(* Logix 5000 AddOnInstructionDefinition export MSQR_Yaskawa; software revision 17.00 *)

TYPE Yaskawa_EIP_Servo :   // Yaskawa SigmaLogic Axis Structure v2.4.0
STRUCT
   O : Yaskawa_OUT_to_Servo;
   I : Yaskawa_IN_from_Servo;
   AOI_SB : Yaskawa_AOI_Status_Bits;
END_STRUCT
END_TYPE

TYPE Yaskawa_OUT_to_Servo :   // Structure of data sent out to the Yaskawa SigmaLogic controller v2.4.0
STRUCT
   b00_ServoOn : BOOL;   // Servo On
   b01_Stop : BOOL;   // Stops All Current Motion in Progress
   b02_Home : BOOL;   // Start Homing Process
   b03_MoveStart1 : BOOL;   // Start Current Motion
   b06_SuperImpose : BOOL;
   b07_ServoAlarmReset : BOOL;   // Servo Alarm Reset
   b08_ControllerAlarmReset : BOOL;   // SigmaLogic Alarm Reset
   b09_MoveStart2 : BOOL;   // Start Second Motion (Blended Move)
   b10_MoveAbort : BOOL;   // Abort Current Move
   b11_MovePause : BOOL;   // Pause Current Move
   b12_SeqPause : BOOL;   // Indexing Sequence Pause
   b13_SeqResume : BOOL;   // Indexing Sequence Resume
   b14_SeqCancel : BOOL;   // Indexing Sequence Cancel
   b15_AbsEncoderReset : BOOL;   // Absolute Encoder Reset
   b16_SeqStart : BOOL;   // Start Indexing Sequence
   b17_SeqEditSpeed : BOOL;   // Enter Edit Speed
   b18_SeqEditDistance : BOOL;   // Enter Distance Edit
   b19_PLSEnable : BOOL;   // Enable PLS execution
   b20_PLSActivateOutput1 : BOOL;   // Activate PLS output1 switch logic
   b21_PLSActivateOutput2 : BOOL;   // Activate PLS output2 switch logic
   b22_PLSActivateOutput3 : BOOL;   // Activate PLS output3 switch logic
   b23_PLSActivateOutput4 : BOOL;   // Activate PLS output4 switch logic
   b24_SetClock : BOOL;   // Set the remote controller clock with data provided by the PLC
   RebootController : BOOL;
   UseExternalEncoder : BOOL;   // Use External Encoder when executing MAHSP_Yaskawa
   b32_HeatbeatAnswer : BOOL;   // Heartbeat Answer
   BrakeBypassRequest : BOOL;
   SetFwdTorqueLimit : BOOL;
   SetRevTorqueLimit : BOOL;
   TorqueLimit : DINT;
   TorqueRamp : DINT;
   HomeMethod : INT;
   HomeSpeed : DINT;
   HomeAccDec : DINT;   // Home Move Acceleration/Deceleration Rate
   HomeBackOffDistance : DINT;
   HomeCreepSpeed : DINT;
   HomeCreepDistanceLimit : DINT;
   HomeCreepTimeLimit : DINT;
   HomeOffsetDistance : DINT;
   HomeOffsetSpeed : DINT;
   HomePostion : DINT;
   HomeTorque : DINT;
   HomeInputNo : DINT;
   HomeApproachTimeLimit : DINT;
   HomeApproachDistLimit : DINT;
   HomeDirection : INT;
   HomeSwitchMode : INT;
   MoveType : INT;
   MoveDirection : INT;
   MoveAccel1 : DINT;
   MoveAccel2 : DINT;
   MoveDecel1 : DINT;
   MoveDecel2 : DINT;
   MoveSpeed1 : DINT;
   MoveSpeed2 : DINT;
   MoveDistance1 : DINT;
   MoveDistance2 : DINT;
   MovePosition1 : DINT;
   MovePosition2 : DINT;
   RegistrationDistance : DINT;
   GearNumerator : DINT;
   GearDenominator : DINT;
   SuperImposeDistance : DINT;
   Resolution : INT;
   RegistrationDirection : INT;
   TuningLevel : INT;
   SequenceStep : INT;   // Staring Sequence Step Number
   SequenceEditStep : INT;   // Sequence Step Number to Edit
   FlagCommandBits1 : DINT;   // Flag Commands. 1..64 are General Flags, Bits 0..31 correspond to Flag 1..32
   FlagCommandBits2 : DINT;   // Flag Commands cont. 1..64 are General Flags, Bits 0..31 correspond to Flag 33..64
   DigitalOutCommandBits : DINT;   // Digital Output commands. Bits 0-7 correspond to CN13 Digital Outputs 0-7, used as Flag 73-80. Bits 8-10 correspond to CN1 Digital Outputs 0-2 used as Flag 88-90"
   SequenceEditSpeed : DINT;
   SequenceEditDistance : DINT;
   FeedRateOverride : INT;
   HSI_Enable : BOOL;
   HSI_MoveMode : BOOL;   // 0=Relative; 1=Moves per Cycle
   HSI_CalcMethod : BOOL;   // 0=Accel/Decel; 1=Time
   HSI_MoveDirection : BOOL;   // 0 = Negative; 1 = Positive
   HSI_TriggerFlag : INT;
   HSI_MovingFlag : INT;
   HSI_DwellingFlag : INT;
   HSI_DoneFlag : INT;
   HSI_MoveType : INT;   // 0=Single; 1=Repeat; 2=Repeat "x" times
   HSI_RepeatNumber : INT;
   HSI_Distance : DINT;
   HSI_Speed : DINT;
   HSI_Accel : DINT;
   HSI_MoveTime : DINT;
   HSI_DwellTime : DINT;
   PLS_OutputFlag1 : INT;
   PLS_OutputFlag2 : INT;
   PLS_OutputFlag3 : INT;
   PLS_OutputFlag4 : INT;
   PLS_OnPosition1 : DINT;
   PLS_OffPosition1 : DINT;
   PLS_OnPosition2 : DINT;
   PLS_OffPosition2 : DINT;
   PLS_OnPosition3 : DINT;
   PLS_OffPosition3 : DINT;
   PLS_OnPosition4 : DINT;
   PLS_OffPosition4 : DINT;
   PLS_OnCompensation1 : INT;
   PLS_OffCompensation1 : INT;
   PLS_OnCompensation2 : INT;
   PLS_OffCompensation2 : INT;
   PLS_OnCompensation3 : INT;
   PLS_OffCompensation3 : INT;
   PLS_OnCompensation4 : INT;
   PLS_OffCompensation4 : INT;
   RTC_Year : INT;
   RTC_Month : INT;
   RTC_Day : INT;
   RTC_Hour : INT;
   RTC_Min : INT;
   RTC_Sec : INT;
   StopDecel : DINT;
   AnalogOutput : INT;   // CN13, AO_01 [mV]
END_STRUCT
END_TYPE

TYPE Yaskawa_AOI_Status_Bits :   // Internal bits used to interlock Yaskawa AOI execution. v2.4.0
STRUCT
   MAM : BOOL;   // Move AOI Active
   MAJ : BOOL;   // Jog AOI Active
   MAB : BOOL;   // Blending AOI Active
   MAG : BOOL;   // Gearing AOI Active
   MAHSP : BOOL;   // Home SetPoint AOI Active
   MAH : BOOL;   // Homing AOI Active
   MSQE : BOOL;   // Sequence Edit AOI Active
   MSQR : BOOL;   // Sequence Run AOI Active
   MHSI : BOOL;   // High Speed Index AOI Active
   MSO : BOOL;   // Servo On
   MSF : BOOL;   // Servo Off
   MAFR : BOOL;   // Fault Reset
   MAS : BOOL;   // Servo Abort
   MTRQ : BOOL;   // Torque Mode Active
   MPLS : BOOL;   // PLS Active
   MCLK : BOOL;   // SetClock Active
   MSTL : BOOL;   // Set Torque Limit Active
   AOI_Permissive : BOOL;   // Permissive to Execute an AOI
END_STRUCT
END_TYPE

TYPE Yaskawa_IN_from_Servo :   // Structure of data coming from the Yaskawa SigmaLogic controller. v2.4.0
STRUCT
   AlarmText : STRING;   // ServoPack Alarm Code plus Text Description
   b00_Heartbeat : BOOL;
   b01_Alarm : BOOL;   // ServoPack Alarm
   b02_Warning : BOOL;   // ServoPack Warning
   b03_Ready : BOOL;   // ServoPack Ready
   b04_Enabled : BOOL;   // ServoPack Enabled ("Servo On")
   b05_StopComplete : BOOL;
   b06_HomeComplete : BOOL;
   b07_HomeBusy : BOOL;
   b08_HomeActive : BOOL;
   b09_HomeAborted : BOOL;
   b10_HomeError : BOOL;
   b11_MoveAbsComplete : BOOL;
   b12_MoveAbsBusy : BOOL;
   b13_MoveAbsActive : BOOL;
   b14_MoveAbsAborted : BOOL;
   b15_MoveAbsError : BOOL;
   b16_MoveRelComplete : BOOL;
   b17_MoveRelBusy : BOOL;
   b18_MoveRelActive : BOOL;
   b19_MoveRelAborted : BOOL;
   b20_MoveRelError : BOOL;
   b21_JogAtSpeed : BOOL;
   b22_JogBusy : BOOL;
   b23_JogActive : BOOL;
   b24_JogAborted : BOOL;
   b25_JogError : BOOL;
   b26_GearInSync : BOOL;
   b27_GearBusy : BOOL;
   b28_GearActive : BOOL;
   b29_GearAborted : BOOL;
   b30_GearError : BOOL;
   b32_MoveSuperComplete : BOOL;
   b33_MoveSuperBusy : BOOL;
   b34_MoveSuperActive : BOOL;
   b35_MoveSuperAborted : BOOL;
   b36_MoveSuperError : BOOL;
   b37_PowerCycleRequired : BOOL;
   b38_MoveBlend1Complete : BOOL;
   b39_MoveBlend1Busy : BOOL;
   b40_MoveBlend1Active : BOOL;
   b41_MoveBlend1Abort : BOOL;
   b42_MoveBlend1Error : BOOL;
   b43_MoveBlend2Complete : BOOL;
   b44_MoveBlend2Busy : BOOL;
   b45_MoveBlend2Active : BOOL;
   b46_MoveBlend2Abort : BOOL;
   b47_MoveBlend2Error : BOOL;
   b48_RegComplete : BOOL;
   b49_RegBusy : BOOL;
   b50_RegActive : BOOL;
   b51_RegAborted : BOOL;
   b52_RegError : BOOL;
   b53_ResetAbsEncoderActive : BOOL;
   b54_ResetAbsEncoderBusy : BOOL;
   b55_ResetAbsEncoderDone : BOOL;
   b56_ResetAbsEncoderError : BOOL;
   b57_SeqRunning : BOOL;
   b58_RegSensorNotReached : BOOL;
   b59_SeqEditError : BOOL;
   b60_SeqEditDone : BOOL;
   b61_TorqueAtTorque : BOOL;
   b62_TorqueBusy : BOOL;
   b63_TorqueActive : BOOL;
   b64_TorqueAborted : BOOL;
   b65_TorqueError : BOOL;
   b66_ControllerAlarm : BOOL;
   b67_ApplicationError : BOOL;
   b68_AxisAtStandStill : BOOL;
   b69_TestModeActive : BOOL;
   b70_ServoParamsOK : BOOL;
   b71_SetFwdTorqueLimitDone : BOOL;
   b72_SetRevTorqueLimitDone : BOOL;
   Position : DINT;
   Speed : DINT;
   Torque : DINT;
   HomeErrorID : INT;
   MoveAbsErrorID : INT;
   MoveRelErrorID : INT;
   JogErrorID : INT;
   GearErrorID : INT;
   MoveSuperErrorID : INT;
   ServoAlarmID : INT;
   ServoWarningID : INT;
   ControllerAlarmID : DINT;
   AxisGenAlarmID : DINT;
   MoveBlend1ErrorID : INT;
   MoveBlend2ErrorID : INT;
   ResetAbsEncoderErrorID : INT;
   FunctionBlockErrorID : INT;
   TorqueErrorID : INT;
   RegErrorID : INT;
   SeqCurrentStep : INT;
   FlagStatusBit1 : DINT;   // Flag Status. 1..64 are General Flags, Bits 0..31 correspond to Flag 1..32
   FlagStatusBit2 : DINT;   // Flag Status cont. 1..64 are General Flags, Bits 0..31 correspond to Flag 33..64
   IOStatusBits : DINT;   // Digital IO Status. Bits 0-7, CN13 Inputs 0-7, Used as Flag 65-72. Bits 8-15, CN13 Outputs 0-7, Used as Flag 73-80. Bits 16-22, CN1 Inputs 0-6, Used as Flag 81-87. Bits 23-25, CN1 Outputs 0-4, Used as Flag 88-92.
   HSI_Moving : BOOL;
   HSI_Dwelling : BOOL;
   HSI_Done : BOOL;
   HSI_Busy : BOOL;
   HSI_Error : BOOL;
   HSI_ErrorCode : INT;
   PLS_Running : BOOL;
   PLS_SwitchStatus1 : BOOL;
   PLS_SwitchStatus2 : BOOL;
   PLS_SwitchStatus3 : BOOL;
   PLS_SwitchStatus4 : BOOL;
   PLS_Busy : BOOL;
   PLS_Error : BOOL;
   PLS_ErrorCode : INT;
   SetClock_Done : BOOL;
   SetClock_Busy : BOOL;
   SetClock_Error : BOOL;
   SetClock_ErrorID : INT;
   SoftwareVersion : DINT;
   FirmwareVersion : DINT;
   CommandedPos : DINT;
   CommandedPosNonCyc : DINT;
   CommandedSpeed : DINT;
   Clock_Year : INT;
   Clock_Month : INT;
   Clock_Day : INT;
   Clock_Hour : INT;
   Clock_Minute : INT;
   Clock_Second : INT;
   AnalogInput : REAL;   // CN13, AI_01 [v]
   BrakeBypassActive : BOOL;
   ForwardTorqueLimit : DINT;
   ReverseTorqueLimit : DINT;
END_STRUCT
END_TYPE

ADD_ON_INSTRUCTION MSQR_Yaskawa   (* revision 2.4 0, vendor Yaskawa America, Inc., ExecuteEnableInFalse *)
// Motion Sequence Run
// Revision note:
// 2.4.0: No functional change
// 2.3.1: No functional change
// 2.3.0: No functional change
// 2.0.0: No functional change.
// 1.2.0: No functional change.
// Initial Release 9/10/2014
// Help:
// This AOI runs a step in the predefined Sequence Table. Other controls are also made available to Pause, Resume or Cancel sequence table execution. Pausing a sequence will also pause motion.
VAR_IN_OUT
   Axis : Yaskawa_EIP_Servo; {required}
END_VAR
VAR_INPUT
   StepNumber : INT; {required}   // Sequence Starting Step #
   SeqPause : BOOL; {required}   // Pause Current Running Sequence
   SeqResume : BOOL; {required}   // Resume Current Running Sequence
   SeqCancel : BOOL; {required}   // Cancel Current Running Sequence
END_VAR
VAR_OUTPUT
   CurrentStep : INT; {visible}   // Indicates the Current Sequence Step #
   EN : BOOL; {visible}   // Function is Executing
   IP : BOOL; {visible}   // Sequence is In Process
   FLT_RDY : BOOL; {visible}   // Conditions are not right for the function to properly complete
   FLT_BSY : BOOL; {visible}   // There is another AOI Active for this Axis
END_VAR
VAR
   AOI_ON_LOCAL : BOOL;
   Seq_ER : BOOL;
END_VAR

ROUTINE EnableInFalse   (* ladder *)
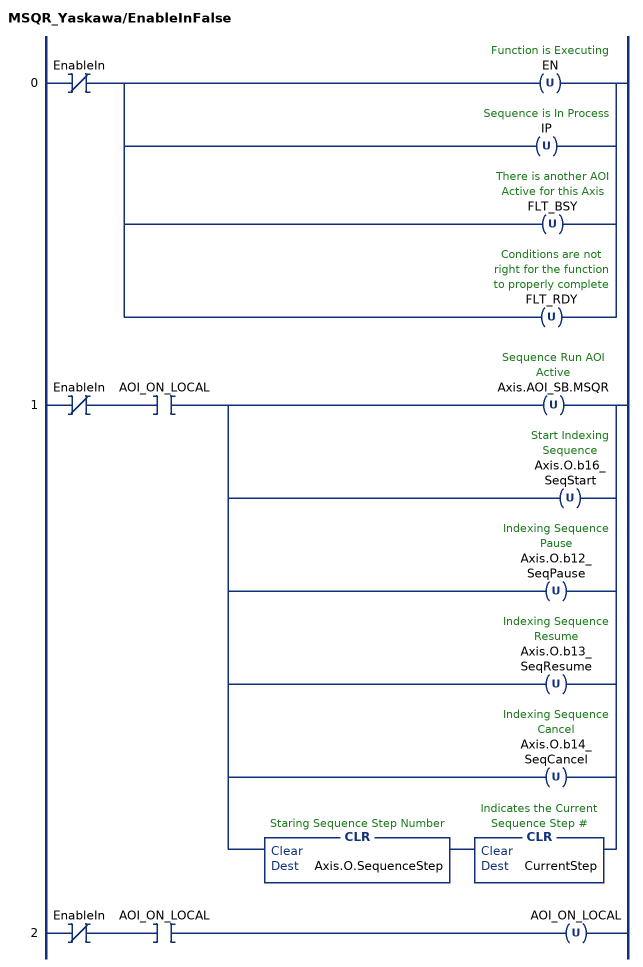
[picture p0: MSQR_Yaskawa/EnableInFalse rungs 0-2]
   0: XIO(EnableIn)[OTU(EN) ,OTU(IP) ,OTU(FLT_BSY) ,OTU(FLT_RDY) ];
   1: XIO(EnableIn)XIC(AOI_ON_LOCAL)[OTU(Axis.AOI_SB.MSQR) ,OTU(Axis.O.b16_SeqStart) ,OTU(Axis.O.b12_SeqPause) ,OTU(Axis.O.b13_SeqResume) ,OTU(Axis.O.b14_SeqCancel) ,CLR(Axis.O.SequenceStep) CLR(CurrentStep) ];
   2: XIO(EnableIn)XIC(AOI_ON_LOCAL)OTU(AOI_ON_LOCAL);
END_ROUTINE

ROUTINE Logic   (* ladder *)
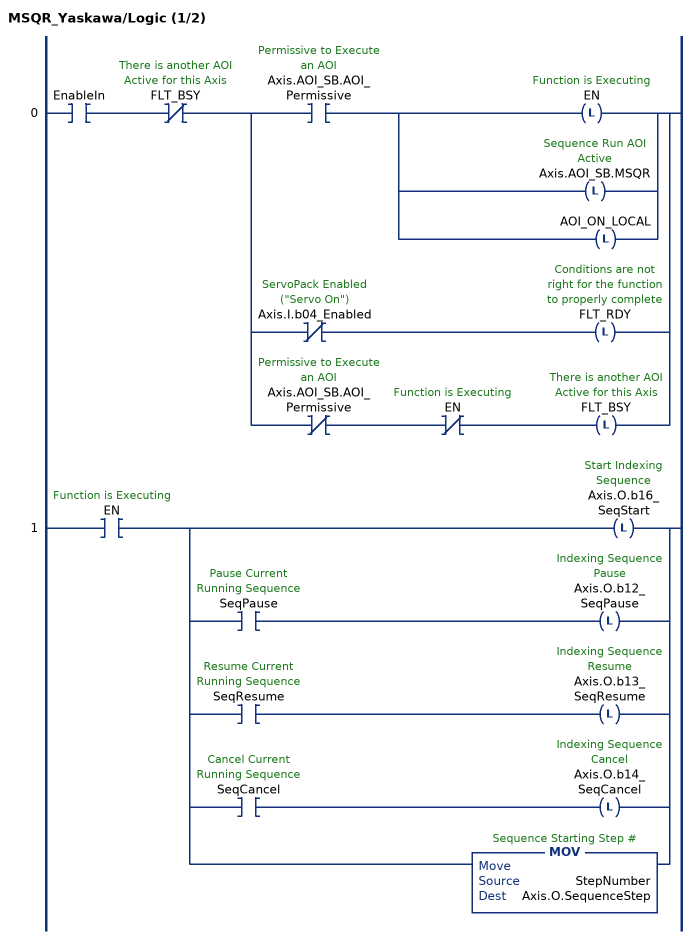
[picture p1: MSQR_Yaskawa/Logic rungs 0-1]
   0: XIC(EnableIn)XIO(FLT_BSY)[XIC(Axis.AOI_SB.AOI_Permissive) [OTL(EN) ,OTL(Axis.AOI_SB.MSQR) ,OTL(AOI_ON_LOCAL) ] ,XIO(Axis.I.b04_Enabled) OTL(FLT_RDY) ,XIO(Axis.AOI_SB.AOI_Permissive) XIO(EN) OTL(FLT_BSY) ];
   1: XIC(EN)[OTL(Axis.O.b16_SeqStart) ,XIC(SeqPause) OTL(Axis.O.b12_SeqPause) ,XIC(SeqResume) OTL(Axis.O.b13_SeqResume) ,XIC(SeqCancel) OTL(Axis.O.b14_SeqCancel) ,MOV(StepNumber,Axis.O.SequenceStep) ];
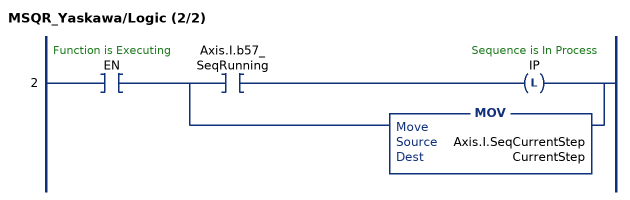
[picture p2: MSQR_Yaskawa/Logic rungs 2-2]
   2: XIC(EN)[XIC(Axis.I.b57_SeqRunning) OTL(IP) ,MOV(Axis.I.SeqCurrentStep,CurrentStep) ];
END_ROUTINE
END_ADD_ON_INSTRUCTION
